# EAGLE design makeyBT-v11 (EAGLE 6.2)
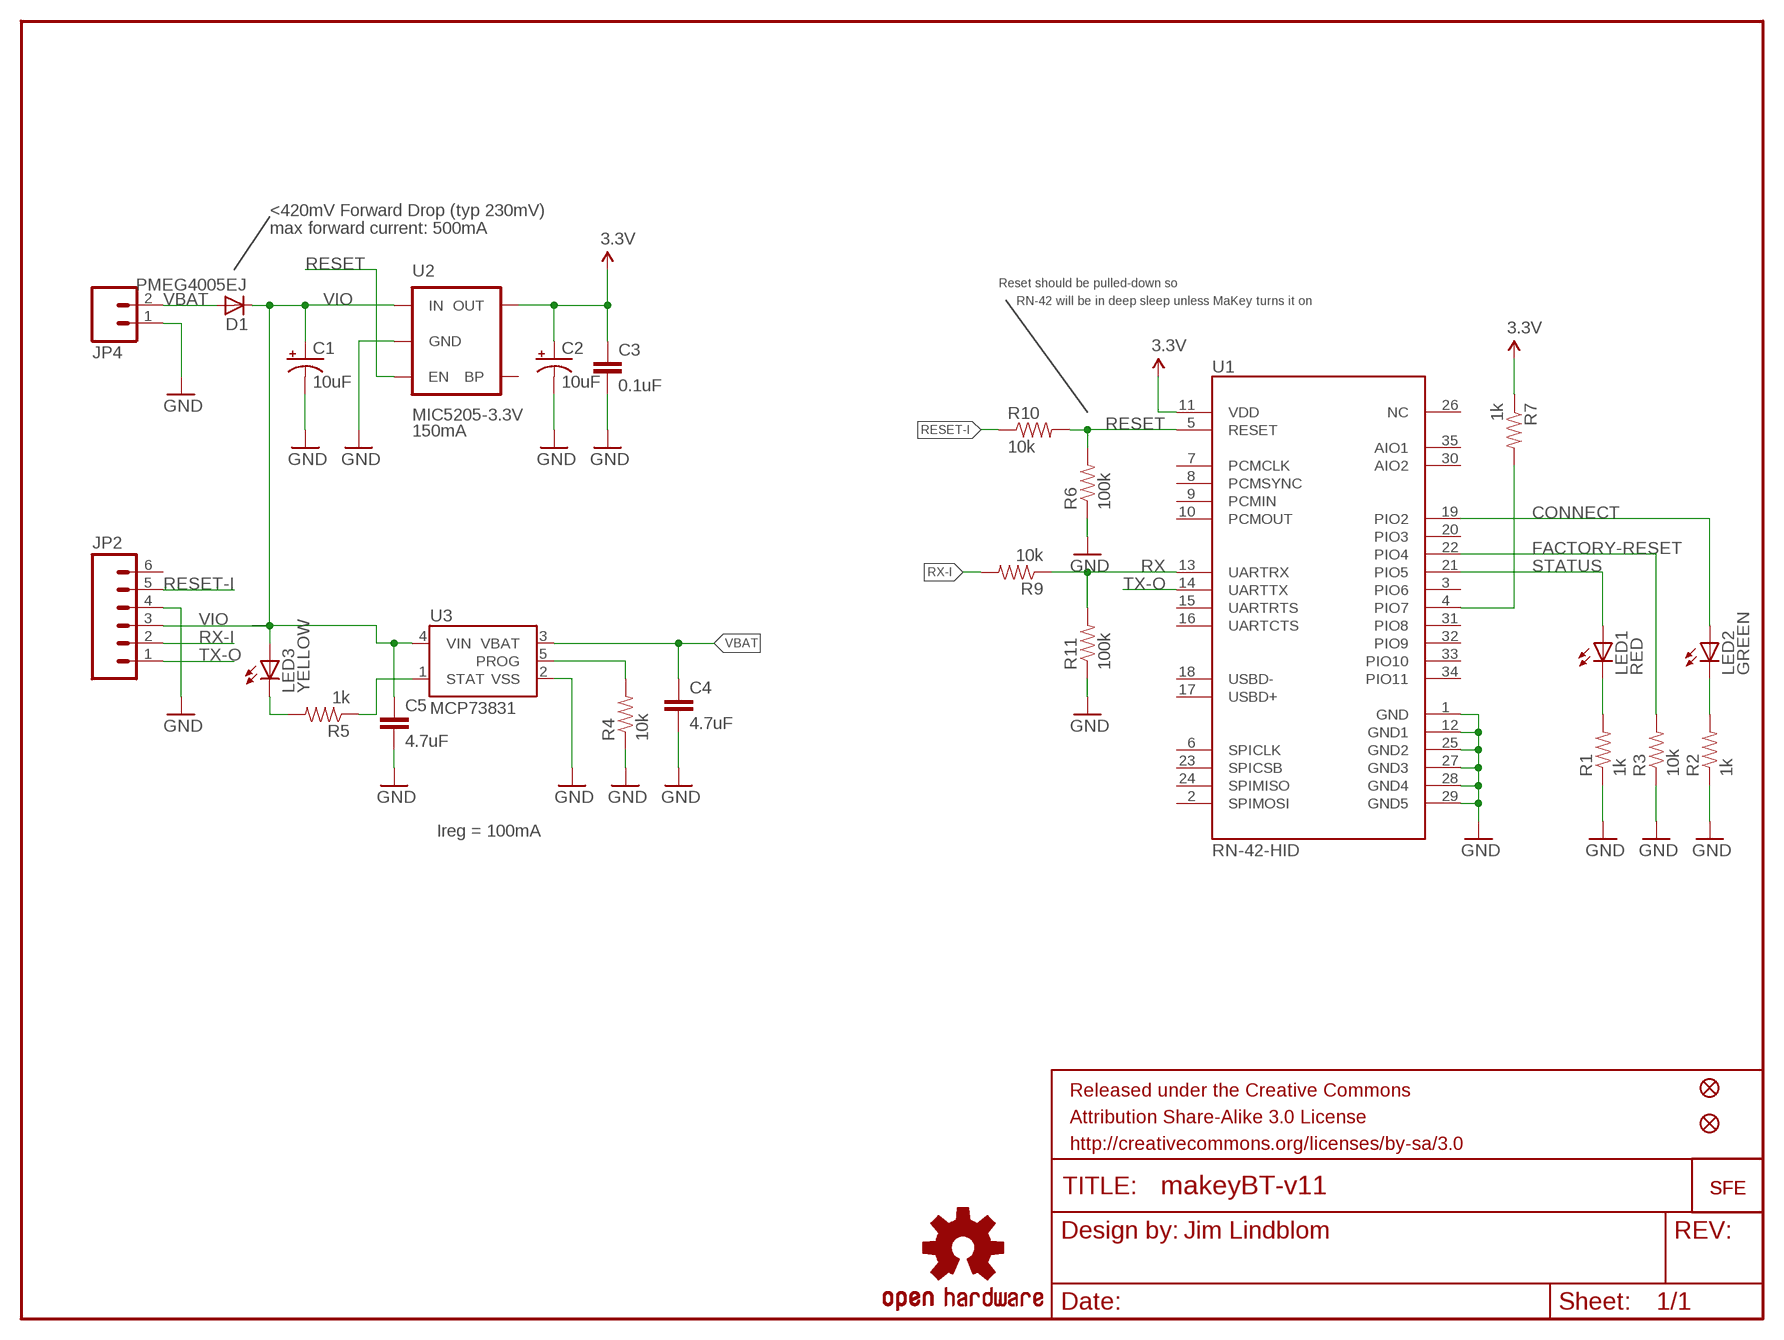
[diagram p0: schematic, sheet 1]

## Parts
C1  10uF  CAP_POL1206  [EIA3216]
C2  10uF  CAP_POL1206  [EIA3216]
C3  0.1uF  CAP0402-CAP  [0402-CAP]
C4  4.7uF  CAP0402-CAP  [0402-CAP]
C5  4.7uF  CAP0402-CAP  [0402-CAP]
D1  PMEG4005EJ  DIODESOD  [SOD-323]
JP1  LOGO-SFESK  [SFE-LOGO-FLAME]
JP2  M06SIP  [1X06]
JP3  LOGO-SFENW2  [SFE-NEW-WEB]
JP4  M02-JST-2MM-SMT  [JST-2-SMD]
JP5  FIDUCIALUFIDUCIAL  [MICRO-FIDUCIAL]
JP6  FIDUCIALUFIDUCIAL  [MICRO-FIDUCIAL]
LED1  RED  LED0603  [LED-0603]
LED2  GREEN  LED0603  [LED-0603]
LED3  YELLOW  LED0603  [LED-0603]
R1  1k  RESISTOR0402-RES  [0402-RES]
R2  1k  RESISTOR0402-RES  [0402-RES]
R3  10k  RESISTOR0402-RES  [0402-RES]
R4  10k  RESISTOR0402-RES  [0402-RES]
R5  1k  RESISTOR0402-RES  [0402-RES]
R6  100k  RESISTOR0402-RES  [0402-RES]
R7  1k  RESISTOR0402-RES  [0402-RES]
R9  10k  RESISTOR0402-RES  [0402-RES]
R10  10k  RESISTOR0402-RES  [0402-RES]
R11  100k  RESISTOR0402-RES  [0402-RES]
U1  RN-42-HID  BLUETOOTH-RN41"  [RN41]
U2  MIC5205-3.3V  V_REG_LDOSMD  [SOT23-5]
U3  MCP73831  [SOT23-5]
U$2  OSHW-LOGOS  [OSHW-LOGO-S]

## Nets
3.3V: C2.A(+) C3.1 R7.1 U1.11(VDD) U2.5(OUT)
CONNECT: LED2.A U1.19(PIO2)
FACTORY-RESET: R3.2 U1.22(PIO4)
GND: C1.C(-) C2.C(-) C3.2 C4.2 C5.2 JP2.4 JP4.1 R1.1 R2.1 R3.1 R4.1 R6.1 R11.1 U1.1(GND) U1.12(GND1) U1.25(GND2) U1.27(GND3) U1.28(GND4) U1.29(GND5) U2.2(GND) U3.2(VSS)
N$1: R7.2 U1.4(PIO7)
N$2: LED1.C R1.2
N$3: LED2.C R2.2
N$4: R4.2 U3.5(PROG)
N$6: R5.1 U3.1(STAT)
N$7: LED3.C R5.2
RESET: R6.2 R10.2 U1.5(RESET) U2.3(EN)
RESET-I: JP2.5 R10.1
RX: R9.1 R11.2 U1.13(UARTRX)
RX-I: JP2.2 R9.2
STATUS: LED1.A U1.21(PIO5)
TX-O: JP2.1 U1.14(UARTTX)
VBAT: C4.1 D1.2(A) JP4.2 U3.3(VBAT)
VIO: C1.A(+) C5.1 D1.1(C) JP2.3 LED3.A U2.1(IN) U3.4(VIN)
Unconnected: JP2.6 U1.2(SPIMOSI) U1.3(PIO6) U1.6(SPICLK) U1.7(PCMCLK) U1.8(PCMSYNC) U1.9(PCMIN) U1.10(PCMOUT) U1.15(UARTRTS) U1.16(UARTCTS) U1.17(USBD+) U1.18(USBD-) U1.20(PIO3) U1.23(SPICSB) U1.24(SPIMISO) U1.26(NC) U1.30(AIO2) U1.31(PIO8) U1.32(PIO9) U1.33(PIO10) U1.34(PIO11) U1.35(AIO1) U2.4(BP)

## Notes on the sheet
- <420mV Forward Drop (typ 230mV)
- max forward current: 500mA
- Reset should be pulled-down so
- RN-42 will be in deep sleep unless MaKey turns it on
- 150mA
- Ireg = 100mA
- Jim Lindblom

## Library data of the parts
C1 C2 = SparkFun-Passives:CAP_POL: Capacitor Polarized
C3-C5 = SparkFun-Passives:CAP: Capacitor
D1 = SparkFun-DiscreteSemi:DIODE: Diode
JP1 JP3 = SparkFun-Aesthetics:LOGO-SFE: Spark Fun Electronics PCB Logo
JP2 = SparkFun-Connectors:M06: Header 6 Standard 6-pin 0.1" header. Use with straight break away headers (SKU : PRT-00116), right angle break away headers (PRT-00553), swiss pins (PRT-00743), machine pins (PRT-00117), and female headers (PRT-00115). Molex polarized connector foot print use with SKU : PRT-08094 with associated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
JP4 = SparkFun-Connectors:M02: Header 2
JP5 JP6 = SparkFun:FIDUCIAL: Fiducial Alignment Points
LED1-LED3 = SparkFun-LED:LED: LEDs
R1-R7 R9-R11 = SparkFun-Passives:RESISTOR: Resistor
U1 = SparkFun-RF:BLUETOOTH-RN41: Bluetooth SMD module
U2 = SparkFun-PowerIC:V_REG_LDO: Voltage Regulator LDO Standard 150mA LDO voltage regulator in SOT-23 layout. Micrel part MIC5205. BP (by-pass) pin is used to lower output noise with 470pF cap.
U3 = SparkFun-PowerIC:MCP73831: Miniature single cell, fully integrated Li-Ion, Li-polymer charge management controller http://ww1.microchip.com/downloads/en/DeviceDoc/21984a.pdf
U$2 = SparkFun-Aesthetics:OSHW-LOGO: Open Source Hardware Logo This logo indicates the piece of hardware it is found on incorporates a OSHW license and/or adheres to the definition of open source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

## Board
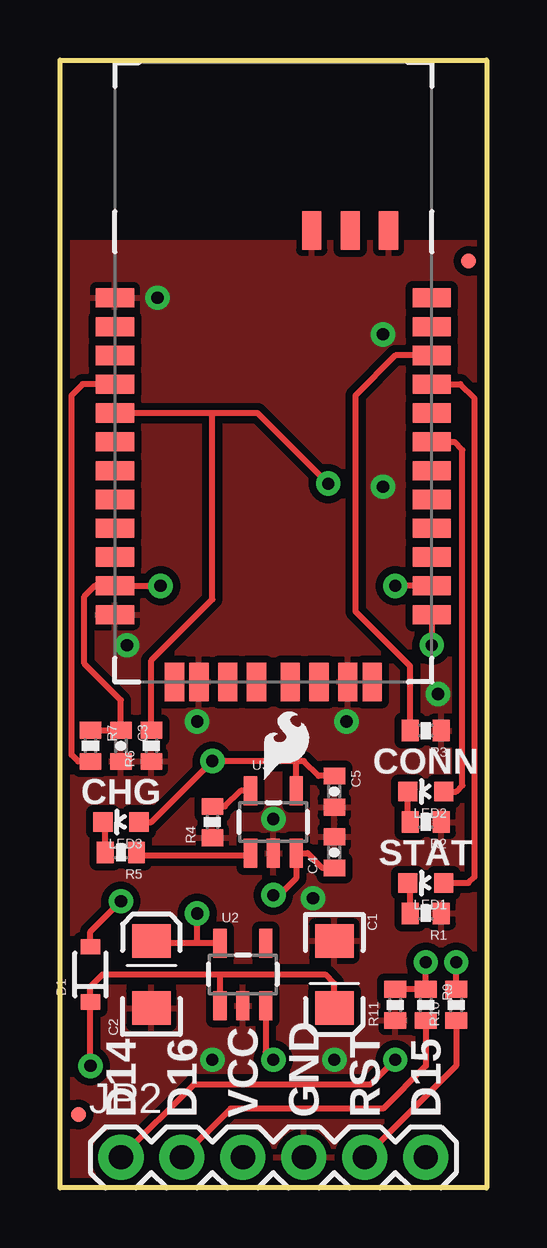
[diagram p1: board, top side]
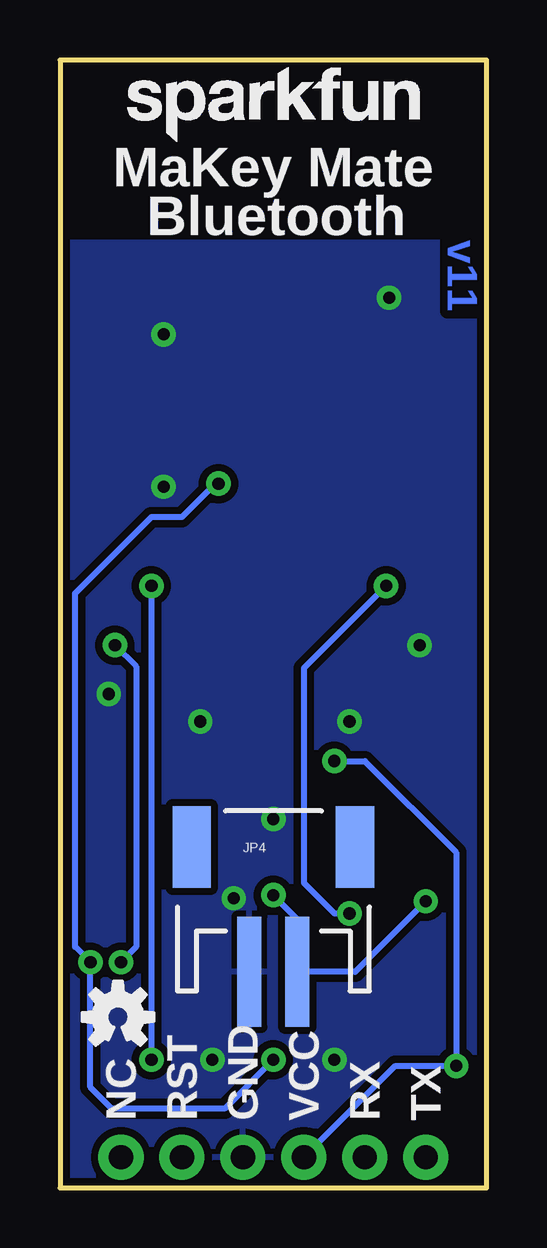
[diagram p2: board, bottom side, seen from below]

Size 17.78 x 46.99 mm. Coordinates in mm from the lower left corner, seen from the top.
Outline: 0,0 0,46.99 17.78,46.99 17.78,0 0,0
Copper layers (1*16): Top 0.035mm / dielectric 1.5mm / Bottom 0.035mm
Design rules: minimum track width 8mil, minimum drill 20mil, track to track 8mil, track to pad 8mil, pad to pad 8mil, via to via 8mil, smd to smd 8mil, copper to edge 8mil, drill to drill 8mil, minimum pad ring 12mil, minimum via ring 10mil, stop-mask expansion 4mil, vias tented up to drill 20mil, thermal gap 10mil

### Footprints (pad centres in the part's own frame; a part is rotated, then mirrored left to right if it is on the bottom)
EIA3216 = smd 1.4 x 1.6: A 1.4,0; C -1.4,0
0402-CAP = smd 0.7 x 0.9: 1 -0.65,0; 2 0.65,0
SOD-323 = smd 0.63 x 0.83: 1 -1.15,0; 2 1.15,0
1X06 = drill 1.016 pad 1.88: 1 0,0; 2 2.54,0; 3 5.08,0; 4 7.62,0; 5 10.16,0; 6 12.7,0
JST-2-SMD = smd 1 x 4.6: 1 -1,-3.7; 2 1,-3.7 | smd 1.6 x 3.4: NC1 -3.4,1.5; NC2 3.4,1.5
MICRO-FIDUCIAL = smd 0.635 x 0.635: 1 0,0
LED-0603 = smd 0.8 x 0.8: A 0,-0.75; C 0,0.75
0402-RES = smd 0.7 x 0.9: 1 -0.65,0; 2 0.65,0
RN41 = smd 0.8 x 1.6: 1 -6.6,-6.6; 2 -5.4,-6.6; 3 -4.2,-6.6; 4 -3,-6.6; 5 -1.8,-6.6; 6 -0.6,-6.6; 7 0.6,-6.6; 8 1.8,-6.6; 9 3,-6.6; 10 4.2,-6.6; 11 5.4,-6.6; 12 6.6,-6.6; 13 6.6,6.6; 14 5.4,6.6; 15 4.2,6.6; 16 3,6.6; 17 1.8,6.6; 18 0.6,6.6; 19 -0.6,6.6; 20 -1.8,6.6; 21 -3,6.6; 22 -4.2,6.6; 23 -5.4,6.6; 24 -6.6,6.6 | smd 1.6 x 0.8: 25 -9.4,4.8; 26 -9.4,3.2; 27 -9.4,1.6; 28 9.4,3.1; 29 9.4,-3.1; 30 9.4,-4.122; 31 9.4,-1.9; 32 9.4,-0.7; 33 9.4,0.7; 34 9.4,1.9; 35 9.4,4.122
SOT23-5 = smd 0.55 x 1.2: 1 -0.95,-1.3; 2 0,-1.3; 3 0.95,-1.3; 4 0.95,1.3; 5 -0.95,1.3

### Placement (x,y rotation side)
C1  11.43,8.89 270 top
C2  3.81,8.89 90 top
C3  2.54,18.41 270 top
C4  11.43,13.97 90 top
C5  11.43,16.51 270 top
D1  1.27,8.89 90 top
JP1  8.51,17.02 0 top
JP2  2.54,1.27 0 top
JP3  14.99,43.56 0 bottom
JP4  8.89,12.7 0 bottom
JP5  0.76,3.05 0 top
JP6  17.02,38.61 0 top
LED1  15.24,12.7 90 top
LED2  15.24,16.51 90 top
LED3  2.54,15.24 90 top
R1  15.24,11.43 180 top
R2  15.24,15.24 180 top
R3  15.24,19.05 180 top
R4  6.35,15.24 90 top
R5  2.54,13.97 180 top
R6  3.81,18.41 90 top
R7  1.27,18.41 270 top
R9  15.24,7.62 270 top
R10  16.51,7.62 90 top
R11  13.97,7.62 90 top
U1  8.89,30.48 270 top
U2  7.62,8.89 0 top
U3  8.89,15.24 0 top
U$2  15.37,7.11 0 bottom

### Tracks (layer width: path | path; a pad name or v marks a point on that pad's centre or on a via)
3.3V  (via drill 0.51)
  Top 0.254: U2.5 5.71,10.19 | v4.19,25.08 U1.11 1.46,25.08 1.02,24.64 1.02,21.84 2.54,20.32 C3.1 R7.1 | 5.71,10.19 3.91,10.19 C2.A | 5.71,10.19 v5.71,11.43
  Bottom 0.254: v4.19,25.08 7.62,21.65 7.62,12.7 6.35,11.43 v5.71,11.43
CONNECT
  Top 0.254: LED2.A 16.51,16.51 16.76,16.76 16.76,30.73 16.42,31.08 U1.19
FACTORY-RESET
  Top 0.254: R3.2 14.59,21.73 12.32,24 12.32,33.02 13.98,34.68 U1.22
GND  (via drill 0.51)
  other vias: 6.35,5.33 11.94,19.43 11.43,5.33 13.46,29.21 8.89,15.37 2.79,22.61 13.46,35.56 10.54,12.06 15.75,20.57 5.71,19.43 4.06,37.08
  pour Top (isolate 0.305): 0,0 0,39.37 17.78,39.37 17.78,0
  pour Bottom (isolate 0.305): 0,0 0,39.37 17.78,39.37 17.78,0
N$1
  Top 0.254: U1.4 0.94,33.48 0.48,33.02 0.48,18.03 0.75,17.77 R7.2
N$2
  Top 0.254: R1.2 14.59,12.6 LED1.C
N$3
  Top 0.254: R2.2 14.49,15.34 LED2.C
N$4
  Top 0.254: R4.2 6.87,15.89 7.52,16.54 U3.5
N$6
  Top 0.254: R5.1 3.32,13.84 7.84,13.84 U3.1
N$7
  Top 0.254: R5.2 1.89,15.14 LED3.C
RESET  (via drill 0.51)
  Top 0.254: 6.35,32.28 8.23,32.28 v11.18,29.34 | 6.35,32.28 U1.5 | 6.35,32.28 6.35,24.51 3.81,21.97 R6.2 | R10.2 v16.51,9.4 | U2.3 8.57,5.65 v8.89,5.33
  Bottom 0.254: v11.18,29.34 11.3,29.34 12.7,27.94 13.97,27.94 17.14,24.77 17.14,10.03 v16.51,9.4 16.51,4.19 15.62,3.3 10.92,3.3 v8.89,5.33
RESET-I
  Top 0.254: R10.1 16.51,5.08 JP2.5
RX  (via drill 0.51)
  Top 0.254: U1.13 v15.49,22.61 | R11.2 R9.1 v15.24,9.4
  Bottom 0.254: v15.49,22.61 14.61,21.73 14.61,10.03 v15.24,9.4
RX-I
  Top 0.254: JP2.2 7.11,3.3 13.46,3.3 15.24,5.08 R9.2
STATUS
  Top 0.254: LED1.A 17.02,12.7 17.27,12.95 17.27,32.89 16.68,33.48 U1.21
TX-O  (via drill 0.51)
  Top 0.254: JP2.1 5.59,4.32 12.95,4.32 v13.97,5.33 | U1.14 v13.97,25.08
  Bottom 0.254: v13.97,25.08 v13.97,5.33
VBAT  (via drill 0.51)
  Top 0.254: C4.1 10.94,13.32 10.32,13.94 U3.3 9.84,12.89 9.14,12.19 v8.89,12.19 | D1.2 1.27,10.67 v2.54,11.94
  Bottom 0.254: v2.54,11.94 5.48,9 JP4.2 7.89,11.19 v8.89,12.19
VIO  (via drill 0.51)
  Top 0.254: 6.64,7.62 U2.1 6.67,8.83 6.73,8.89 | 6.73,8.89 1.78,8.89 1.27,8.38 D1.1 v1.27,5.08 | 6.73,8.89 11.05,8.89 11.43,8.51 C1.A | C5.1 10.78,17.16 10.16,17.78 9.78,17.78 | 9.78,17.78 v6.35,17.78 3.81,15.24 LED3.A | U3.4 9.84,17.72 9.78,17.78
  Bottom 0.254: JP2.3 3.81,5.08 v1.27,5.08 1.27,13.97 5.08,17.78 v6.35,17.78

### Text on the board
Bottom: v11
tPlace: CONN | CHG | STAT | D14 | D16 | VCC | GND | RST | D15
bPlace: MaKey Mate | Bluetooth | TX | RX | VCC | GND | RST | NC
